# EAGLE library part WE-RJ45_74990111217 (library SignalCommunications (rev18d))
Order Code 74990111217 Design THT xBase-T 10/100 Base-T Ports 1x1 Application Standard HPLE Tab Position Up LED (Left-Right) yellow-green EMI Fingers YES Details see: http://katalog.we-online.de/en/pbs/WE-LAN-RJ45/74990111217 Created by Yingchun Shan 2014-07-10 2016 (C) Würth Elektronik
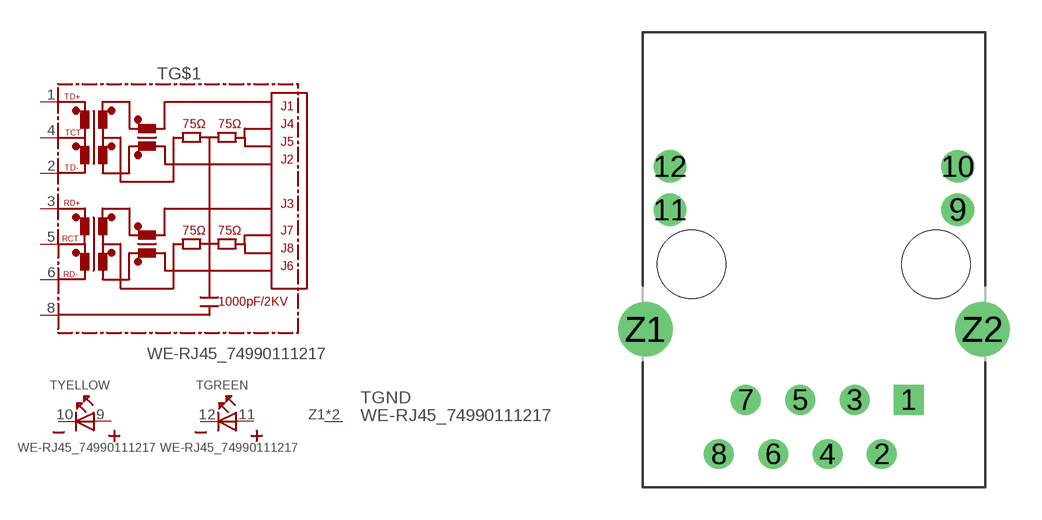
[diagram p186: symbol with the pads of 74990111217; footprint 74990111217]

Designator prefix T; gates G$1=74990111217 GND=GNDPIN YELLOW=LED-2PIN GREEN=LED-2PIN

## WE-RJ45_74990111217  [74990111217]
1  G$1:TD+
2  G$1:TD-
3  G$1:RD+
4  G$1:TCT
5  G$1:RCT
6  G$1:RD-
8  G$1:8
9  YELLOW:A  pas
10  YELLOW:K  pas
11  GREEN:A  pas
12  GREEN:K  pas
Z1  GND:GND  pwr
Z2  GND:GND  pwr

## Footprint 74990111217 (pad centres in mm)
drill 0.89 square: 1 4.44,-6.35
drill 0.89: 2 3.18,-8.89; 3 1.9,-6.35; 4 0.64,-8.89; 5 -0.64,-6.35; 6 -1.9,-8.89; 7 -3.18,-6.35; 8 -4.44,-8.89
drill 1.02: 9 6.725,2.54; 10 6.725,4.57; 11 -6.725,2.54; 12 -6.725,4.57
drill 1.7: Z1 -7.875,-3.05; Z2 7.875,-3.05
hole 3.2 at -5.715,0
hole 3.2 at 5.715,0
